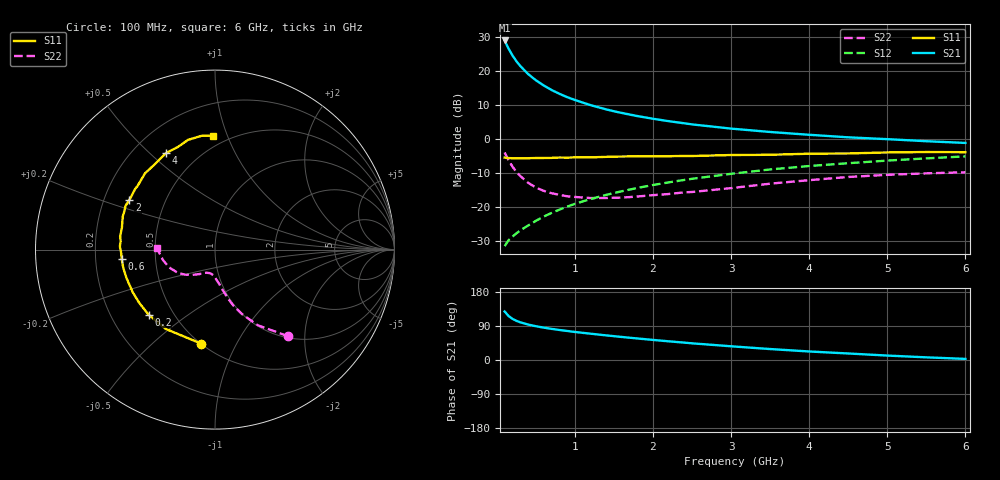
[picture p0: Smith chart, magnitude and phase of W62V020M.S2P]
! SIEMENS Small Signal Semiconductors
! BFR193W
! Si NPN RF Bipolar Junction Transistor in SOT323
! VCE = 2 V  IC = 20 mA
! Common Emitter S-Parameters:  September  1992
# GHz  S  MA  R  50
!  f  S11  S21  S12  S22
! GHz  MAG  ANG  MAG  ANG  MAG  ANG  MAG  ANG
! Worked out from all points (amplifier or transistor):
!   28 points, 100 MHz to 6 GHz, reference 50 ohm
!   highest |S21| = 28.9 dB at 100 MHz (marker M1)
!   |S21| within 3 dB of that: start of sweep to 165.5 MHz
!   unconditionally stable (mu >= 1): 702.9 MHz to 2.567 GHz
!   at 300 MHz: K = 0.77, MSG = 24.1 dB, |S12| = -26.9 dB
!   at 1.5 GHz: K = 1.04, MAG = 10.8 dB, |S12| = -15.9 dB
!   at 6 GHz: K = 0.92, MSG = 2.0 dB, |S12| = -5.2 dB
!   lowest NFmin = 1.40 dB at 450 MHz
!   S11 on the Smith chart (normalised r, x): 100 MHz: 0.50, -0.73; 200 MHz: 0.36, -0.36; 600 MHz: 0.31, -0.05; 2 GHz: 0.31, +0.25; 4 GHz: 0.33, +0.56; 6 GHz: 0.42, +0.89
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0.1  0.5294 -98.4  27.71 128.1  0.0265 57.1  0.6306 -49.9
0.15  0.5202 -121.7  21.06 116.3  0.0323 54.4  0.4844 -60.5
0.2  0.5181 -135.6  16.75 108.6  0.0366 54.2  0.3918 -67.1
0.25  0.5159 -145.0  13.79 103.5  0.0407 55.3  0.326 -72.0
0.3  0.5162 -152.2  11.71 99.5  0.0451 57.0  0.284 -74.9
0.4  0.5181 -162.2  8.932 93.6  0.0532 60.0  0.2262 -79.6
0.5  0.5211 -168.8  7.222 89.2  0.0624 62.6  0.1923 -83.0
0.6  0.5223 -174.1  6.06 85.5  0.072 64.1  0.172 -86.6
0.7  0.5236 -178.3  5.2 82.2  0.0814 65.3  0.1587 -89.1
0.8  0.5304 178.1  4.581 79.3  0.0909 66.3  0.1503 -91.9
0.9  0.5278 174.9  4.082 76.6  0.101 66.8  0.1431 -93.9
1  0.5338 172.0  3.707 74.0  0.1107 67.1  0.1399 -96.1
1.2  0.5327 166.7  3.113 69.4  0.1303 67.1  0.1347 -101.5
1.5  0.5465 160.0  2.532 62.9  0.1597 66.4  0.1363 -108.1
2  0.5516 149.8  1.965 53.0  0.2094 64.2  0.1486 -117.0
2.2  0.5542 145.9  1.812 49.3  0.2288 63.0  0.1544 -119.8
3  0.5768 132.5  1.409 36.2  0.3059 57.2  0.1885 -131.6
3.5  0.5816 125.5  1.257 28.9  0.3542 53.0  0.219 -140.4
4  0.6031 116.8  1.143 22.5  0.398 48.6  0.2466 -148.9
4.5  0.6082 109.8  1.049 17.2  0.4375 44.3  0.2747 -159.0
5.5  0.6383 96.8  0.92 7.0  0.5149 35.7  0.3106 -176.4
6  0.6348 90.9  0.868 2.9  0.5509 31.1  0.322 178.2
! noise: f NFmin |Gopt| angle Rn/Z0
0.45  1.4  0.3  160  0.1
0.9  1.45  0.34  172  0.11
1.8  2.2  0.56  -148  0.2
